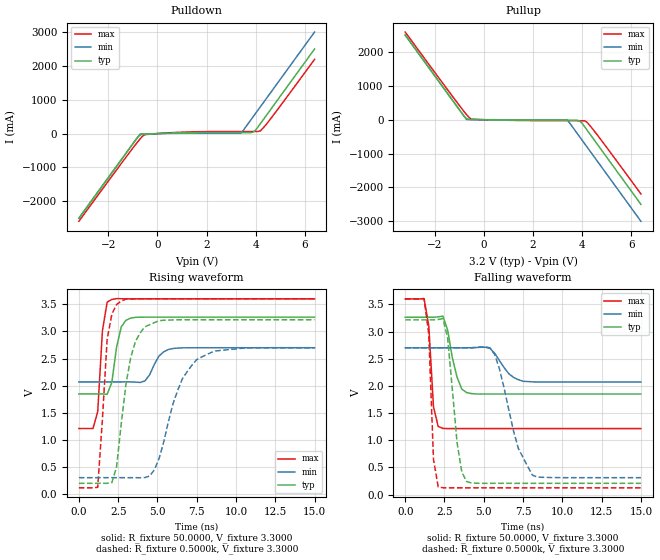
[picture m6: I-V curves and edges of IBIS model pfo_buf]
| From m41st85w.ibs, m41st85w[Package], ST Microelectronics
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|   Model pfo_buf
[Model]   pfo_buf
Model_type   Output
Polarity   Non-Inverting
Vmeas =   1.5000V
Cref =  50.0000pF
Rref =   0.3330k
Vref =   1.7300V
C_comp   7.8500pF   7.4800pF   8.3000pF
[Temperature Range]   27.0000   85.0000   -40.0000
[Voltage Range]   3.2000V   2.7000V   3.6000V
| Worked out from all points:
|   slope of the pulldown table from 0 to 0.48 V, typ, clamps not added: 36.6 ohm
|   slope of the pullup table from 0 to 0.48 V, typ, clamps not added: 94.9 ohm
|   rising waveform, R_fixture 50.0000, V_fixture 3.3000: 20-80 % time 484ps typ, 707ps min, 329ps max; typ from 1.85 V to 3.26 V
|   rising waveform, R_fixture 0.5000k, V_fixture 3.3000: 20-80 % time 881ps typ, 1.58ns min, 469ps max; typ from 0.206 V to 3.21 V
|   falling waveform, R_fixture 50.0000, V_fixture 3.3000: 20-80 % time 608ps typ, 949ps min, 295ps max; typ from 3.26 V to 1.85 V
|   falling waveform, R_fixture 0.5000k, V_fixture 3.3000: 20-80 % time 597ps typ, 1.24ns min, 271ps max; typ from 3.21 V to 0.206 V
[Pulldown]
| voltage   I(typ)   I(min)   I(max)
-3.2V     -2.5A      -2.5A      -2.589A
-900mV    -200mA     -200mA     -332.4mA
-700mV    -40.4mA    -13.31mA   -150.9mA
-500mV    -15.73mA   -8.995mA   -29.69mA
200mV     6.015mA    3.23mA     11mA
1.5V      27.52mA    12.26mA    53.29mA
3.4V      30.47mA    13.72mA    62.33mA
3.9V      46.06mA    500mA      62.93mA
4V        105.2mA    600mA      63.05mA
4.2V      300mA      800mA      84.98mA
4.8V      900mA      1.4A       619.9mA
6.4V      2.5A       3A         2.193A
[Pullup]
| voltage   I(typ)   I(min)   I(max)
-3.2V     2.5A       2.5A       2.589A
-800mV    100mA      100mA      238mA
-700mV    33.38mA    5.779mA    148.1mA
-500mV    6.248mA    3.443mA    15.41mA
-400mV    4.956mA    2.743mA    8.595mA
3.4V      -14.64mA   -7.302mA   -29.56mA
3.9V      -37.09mA   -500mA     -30.29mA
4V        -101.6mA   -600mA     -30.44mA
4.1V      -200mA     -700mA     -32.65mA
4.2V      -300mA     -800mA     -72.2mA
4.8V      -900mA     -1.4A      -618.8mA
6.4V      -2.5A      -3A        -2.193A
[Ramp]
| variable   typ   min   max
dV/dt_r   1.4713/1.0333n   0.9542/1.9812n   1.8636/0.5683n
dV/dt_f   1.7403/0.5718n   1.3401/1.2255n   2.0486/0.3026n
R_load = 0.3330k
[Rising Waveform]
R_fixture = 50.0000
V_fixture = 3.3000
V_fixture_min = 2.7000
V_fixture_max = 3.6000
| time   V(typ)   V(min)   V(max)
0s        1.85V      2.072V     1.213V
900ps     1.85V      2.072V     1.216V
1.2ns     1.85V      2.072V     1.524V
1.5ns     1.85V      2.072V     3.013V
1.8ns     1.843V     2.072V     3.539V
2.1ns     2.065V     2.072V     3.588V
2.7ns     3.086V     2.072V     3.602V
3.3ns     3.246V     2.072V     3.599V
6ns       3.263V     2.686V     3.6V
15ns      3.263V     2.7V       3.6V
[Rising Waveform]
R_fixture = 0.5000k
V_fixture = 3.3000
V_fixture_min = 2.7000
V_fixture_max = 3.6000
| time   V(typ)   V(min)   V(max)
0s        206.2mV    310.1mV    123.5mV
1.2ns     206.2mV    310.1mV    132.8mV
1.8ns     205.4mV    310.1mV    2.854V
2.4ns     508mV      310.1mV    3.496V
3.3ns     2.522V     310.2mV    3.597V
4.2ns     3.085V     311.4mV    3.6V
4.8ns     3.161V     450.8mV    3.6V
6.3ns     3.214V     1.924V     3.6V
7.5ns     3.215V     2.482V     3.6V
15ns      3.215V     2.7V       3.6V
[Falling Waveform]
R_fixture = 50.0000
V_fixture = 3.3000
V_fixture_min = 2.7000
V_fixture_max = 3.6000
| time   V(typ)   V(min)   V(max)
0s        3.263V     2.7V       3.6V
1.2ns     3.263V     2.7V       3.605V
1.5ns     3.263V     2.7V       3.106V
1.8ns     3.263V     2.7V       1.614V
2.1ns     3.269V     2.7V       1.252V
2.4ns     3.281V     2.7V       1.216V
3.3ns     2.158V     2.7V       1.214V
3.9ns     1.876V     2.7V       1.213V
7.5ns     1.85V      2.084V     1.213V
15ns      1.85V      2.072V     1.213V
[Falling Waveform]
R_fixture = 0.5000k
V_fixture = 3.3000
V_fixture_min = 2.7000
V_fixture_max = 3.6000
| time   V(typ)   V(min)   V(max)
0s        3.215V     2.7V       3.6V
1.2ns     3.215V     2.7V       3.606V
1.5ns     3.215V     2.7V       2.953V
1.8ns     3.214V     2.7V       647.8mV
2.1ns     3.222V     2.7V       141.2mV
2.7ns     2.885V     2.7V       123mV
3.9ns     241mV      2.7V       123.5mV
5.7ns     206.3mV    2.573V     123.6mV
8.1ns     206.1mV    356mV      123.4mV
15ns      206.1mV    310.1mV    123.5mV
